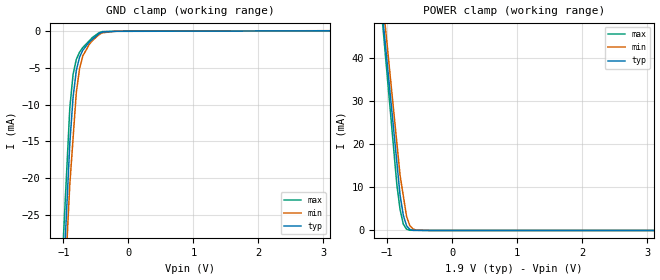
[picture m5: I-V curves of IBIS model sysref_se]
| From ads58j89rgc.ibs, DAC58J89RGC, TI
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[Model] sysref_se
Model_type Input
Vinl = 400.000mV
Vinh = 1.2000V
C_comp 1.06000pF 1.03000pF 1.09000pF
| variable typ   min   max
[Voltage Range] 1.90000V 1.80000V 2.00000V
[POWER Clamp Reference] 1.90000V 1.80000V 2.00000V
[GND Clamp Reference] 0.00000V 0.00000V 0.00000V
[Temperature Range]   25   85   -40
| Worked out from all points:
|   GND clamp passes 1 mA (typ) near -0.54 V on its own axis
|   POWER clamp passes 1 mA (typ) near -0.69 V on its own axis
[GND Clamp]
-1.9V     -202mA     -199.7mA   -190.7mA
-900mV    -15.31mA   -20.88mA   -10.49mA
-850mV    -9.052mA   -14.63mA   -5.918mA
-800mV    -5.365mA   -8.379mA   -3.854mA
-750mV    -3.542mA   -5.116mA   -2.874mA
-700mV    -2.599mA   -3.384mA   -2.238mA
-600mV    -1.484mA   -1.798mA   -1.315mA
-550mV    -1.099mA   -1.266mA   -854.1uA
-450mV    -330.8uA   -483.8uA   -217.7uA
-400mV    -127.2uA   -227.1uA   -66.07uA
-200mV    -33.49uA   -21.54uA   -12.92uA
3.8V      64.31uA    74.44uA    39.99uA
[POWER Clamp]
-1.9V     178.2mA    180.2mA    189.8mA
-950mV    31.4mA     35.64mA    27.8mA
-850mV    15.95mA    20.43mA    10.75mA
-800mV    8.222mA    12.82mA    4.883mA
-750mV    3.548mA    8.042mA    1.473mA
-700mV    1.097mA    3.265mA    304uA
-650mV    238.3uA    1.128mA    47.87uA
-600mV    37.43uA    347uA      41.49uA
-550mV    31.19uA    64.51uA    35.11uA
3.8V      0A         0A         0A
